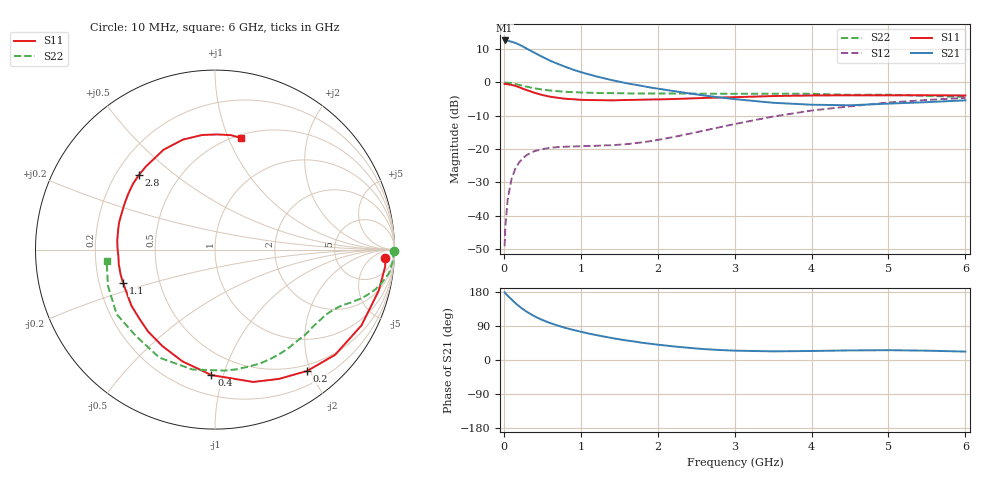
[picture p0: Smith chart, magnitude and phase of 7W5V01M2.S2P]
! Infineon Technologies  Discrete & RF Semiconductors
! BFS17W
! Si NPN RF Bipolar Junction Transistor in SOT323
! VCE = 5 V  IC = 1.2 mA
! Common Emitter S-Parameters:  August  1999
# GHz  S  MA  R  50
!  f  S11  S21  S12  S22
! GHz  MAG  ANG  MAG  ANG  MAG  ANG  MAG  ANG
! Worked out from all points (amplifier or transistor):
!   36 points, 10 MHz to 6 GHz, reference 50 ohm
!   highest |S21| = 12.6 dB at 10 MHz (marker M1)
!   |S21| within 3 dB of that: start of sweep to 342.3 MHz
!   unconditionally stable (mu >= 1): 993.1 MHz to end of sweep
!   at 250 MHz: K = 0.28, MSG = 16.7 dB, |S12| = -22.7 dB
!   at 1.4 GHz: K = 1.27, MAG = 6.6 dB, |S12| = -18.8 dB
!   at 6 GHz: K = 1.09, MAG = -2.2 dB, |S12| = -4.6 dB
!   S11 on the Smith chart (normalised r, x): 10 MHz: 21, -20; 200 MHz: 0.40, -1.95; 400 MHz: 0.33, -0.91; 1.1 GHz: 0.30, -0.16; 2.8 GHz: 0.29, +0.38; 6 GHz: 0.53, +1.11
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0.01  0.9504 -2.7  4.271 178.6  0.0035 84.2  0.9999 -0.3
0.02  0.9527 -5.8  4.246 176.0  0.0069 89.4  0.9951 -1.5
0.05  0.9404 -14.1  4.243 169.6  0.0177 82.4  0.9916 -4.0
0.1  0.9188 -27.4  4.081 160.0  0.0357 74.9  0.9777 -7.8
0.15  0.8897 -41.2  3.926 150.2  0.051 67.0  0.9489 -11.1
0.2  0.8489 -52.8  3.697 141.7  0.0636 61.6  0.921 -13.9
0.25  0.8037 -63.7  3.458 133.9  0.0734 55.7  0.8906 -16.2
0.3  0.7675 -73.9  3.211 127.0  0.0822 51.6  0.8645 -18.1
0.4  0.6994 -91.6  2.786 115.1  0.0935 44.8  0.8173 -21.0
0.5  0.6487 -106.2  2.423 105.7  0.0998 40.3  0.7822 -23.1
0.6  0.6123 -118.6  2.128 97.7  0.1048 37.6  0.7582 -25.0
0.7  0.5894 -129.3  1.905 90.9  0.1073 36.1  0.7402 -26.9
0.9  0.5607 -146.2  1.557 79.5  0.1096 34.8  0.7146 -30.7
1.1  0.545 -159.8  1.328 69.9  0.1118 36.4  0.7019 -34.9
1.4  0.5395 -175.9  1.087 58.2  0.1145 41.4  0.6921 -41.8
1.6  0.5467 175.0  0.971 51.4  0.119 46.2  0.6858 -46.7
2.2  0.5643 153.6  0.745 36.0  0.1514 60.4  0.6831 -62.8
2.8  0.5939 135.5  0.598 26.4  0.2124 66.4  0.6775 -80.1
3.5  0.6258 117.3  0.496 22.8  0.3082 64.5  0.6796 -100.7
4.5  0.6425 96.4  0.455 25.3  0.4387 52.3  0.6523 -132.7
5.5  0.6439 82.0  0.507 24.6  0.5463 38.9  0.6296 -161.3
6  0.638 76.8  0.54 22.2  0.5875 32.5  0.6073 -174.0
